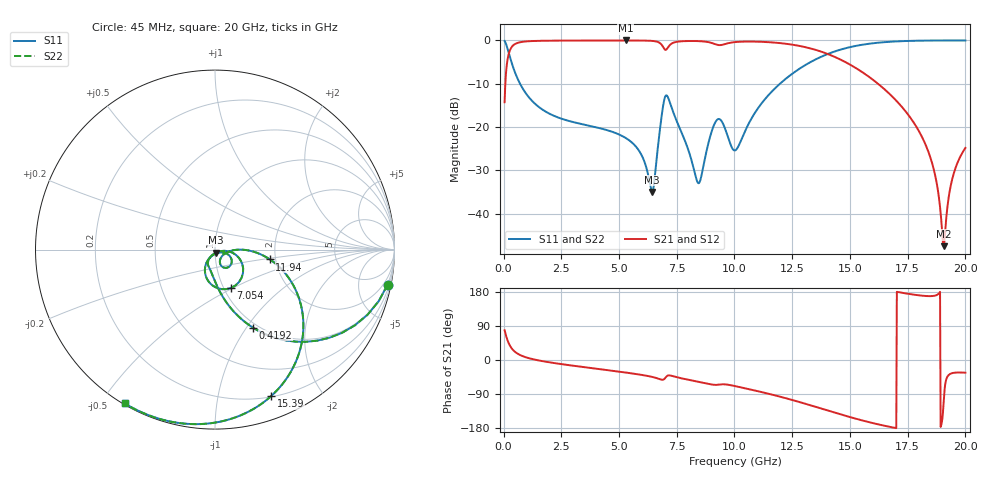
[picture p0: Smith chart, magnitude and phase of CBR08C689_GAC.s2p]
! S-parameter model data by Modelithics Inc.  support@modelithics.com 813-866-6335  Tampa FL USA
! S-Parameter data specifications:
! Substrate: 20-mil Rogers 4350B, substrate thickness, H=0.508mm, Dielectric constant, Er=3.75
! PCB Mounting Pad Footprint: Pad width, PadW=1.45mm , Pad length, PadL=1mm , Pad gap, PadG (edge-to-edge)=0.6mm , Reference planes=2.6mm apart
#  GHz  S  MA  R 50
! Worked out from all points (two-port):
!   801 points, 45 MHz to 20 GHz, reference 50 ohm
!   highest |S21| = -0.06 dB at 5.283 GHz (marker M1); lowest = -47.5 dB at 19.05 GHz (marker M2)
!   |S21| within 3 dB of the highest: 228.1 MHz to 13.98 GHz (13.75 GHz wide, 194 % of centre)
!   lowest |S11| = -35.0 dB at 6.431 GHz (marker M3), VSWR 1.04, Z = 50.6 - j1.68 ohm
!   |S11| at or under -10 dB: 709.8 MHz to 11.98 GHz (11.27 GHz wide, 178 % of centre)
!   |S22| runs from -35.0 to 0.0 dB; largest |S21 - S12| = 0
!   S11 on the Smith chart (normalised r, x): 45 MHz: 0.95, -9.89; 419.2 MHz: 0.95, -1.07; 7.054 GHz: 1.08, -0.49; 11.94 GHz: 1.86, -0.23; 15.39 GHz: 0.21, -1.43; 20 GHz: 0.00, -0.57
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0.045  0.9812 -11.4  0.1928 78.6  0.1928 78.6  0.9812 -11.4
0.219606  0.7227 -45.3  0.6907 44.7  0.6907 44.7  0.7227 -45.3
0.419156  0.4836 -64.0  0.8747 25.9  0.8747 25.9  0.4836 -64.0
1.466794  0.175 -90.2  0.9834 -0.5  0.9834 -0.5  0.175 -90.2
3.387462  0.1078 -107.2  0.9921 -18.1  0.9921 -18.1  0.1078 -107.2
5.283188  0.07473 -120.6  0.9934 -33.0  0.9934 -33.0  0.07473 -120.6
5.956669  0.04838 -121.9  0.9921 -39.1  0.9921 -39.1  0.04838 -121.9
6.4306  0.01782 -68.5  0.983 -44.5  0.983 -44.5  0.01782 -68.5
6.704981  0.06596 -6.9  0.9496 -49.3  0.9496 -49.3  0.06596 -6.9
7.054194  0.2314 -67.7  0.7834 -43.6  0.7834 -43.6  0.2314 -67.7
8.4261  0.02252 -75.2  0.9777 -57.3  0.9777 -57.3  0.02252 -75.2
9.249244  0.1211 -42.1  0.8867 -65.5  0.8867 -65.5  0.1211 -42.1
10.0225  0.05359 -39.1  0.9521 -68.8  0.9521 -68.8  0.05359 -39.1
11.94317  0.3106 -10.1  0.9288 -96.3  0.9288 -96.3  0.3106 -10.1
13.36496  0.5734 -33.2  0.7951 -120.9  0.7951 -120.9  0.5734 -33.2
15.38541  0.8739 -69.0  0.4549 -157.1  0.4549 -157.1  0.8739 -69.0
16.68248  0.9586 -88.1  0.245 -175.9  0.245 -175.9  0.9586 -88.1
18.35371  0.9917 -106.8  0.05548 168.7  0.05548 168.7  0.9917 -106.8
18.72787  0.9935 -110.2  0.02475 170.6  0.02475 170.6  0.9935 -110.2
19.05214  0.9943 -113.0  0.00421 -117.1  0.00421 -117.1  0.9943 -113.0
19.45124  0.9944 -116.3  0.0263 -34.4  0.0263 -34.4  0.9944 -116.3
20  0.9937 -120.4  0.05726 -33.5  0.05726 -33.5  0.9937 -120.4
